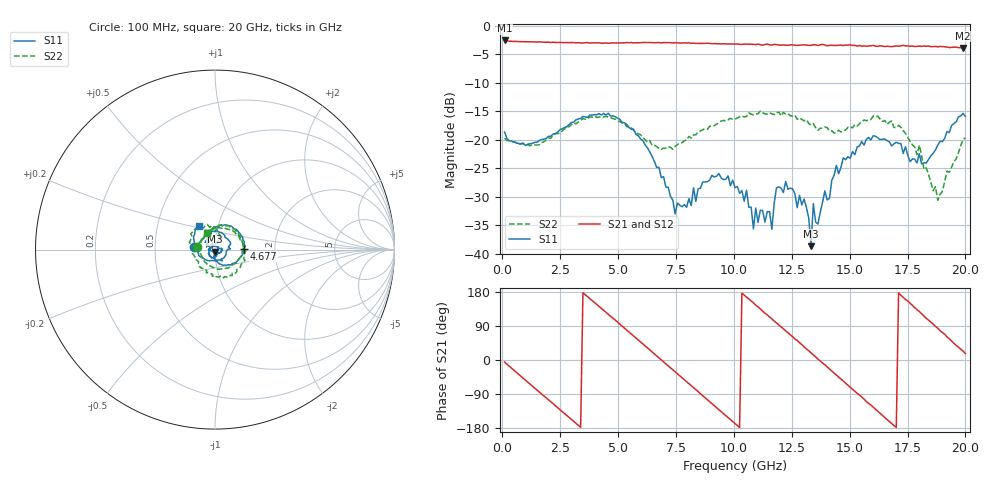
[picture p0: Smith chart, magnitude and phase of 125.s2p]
!Agilent Technologies,N5230C,MY49001569,A.09.33.09
!Agilent N5230C: A.09.33.09
!Date: Tuesday, July 28, 2015 18:46:54
!Correction: S11(Full 2 Port(1,2))
!S21(Full 2 Port(1,2))
!S12(Full 2 Port(1,2))
!S22(Full 2 Port(1,2))
!S2P File: Measurements: S11, S21, S12, S22:
# Hz S  dB  R 50
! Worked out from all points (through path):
!   201 points, 100 MHz to 20 GHz, reference 50 ohm
!   highest |S21| = -2.59 dB at 100 MHz (marker M1); lowest = -3.9 dB at 19.9 GHz (marker M2)
!   group delay of S21, straight-line fit = 147 ps
!   lowest |S11| = -38.7 dB at 13.33 GHz (marker M3), VSWR 1.02, Z = 49.9 - j1.15 ohm
!   |S11| at or under -10 dB: start of sweep to end of sweep
!   |S22| runs from -30.6 to -15.0 dB; largest |S21 - S12| = 0.018
!   S11 on the Smith chart (normalised r, x): 100 MHz: 0.79, +0.03; 4.677 GHz: 1.38, +0.01; 20 GHz: 0.81, +0.22
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1e8  -18.66 172.0  -2.59 -5.4  -2.63 -6.0  -19.74 172.7
1.692e9  -19.97 119.7  -2.88 -89.5  -2.88 -89.4  -20.51 123.6
3.483e9  -15.94 54.6  -3.03 177.5  -3.02 177.6  -16.30 60.3
4.677e9  -15.86 1.8  -3.06 115.4  -3.01 115.7  -16.12 -0.1
5.5725e9  -18.20 -39.7  -2.96 68.9  -2.99 68.9  -17.95 -53.9
6.7665e9  -24.86 -85.3  -2.97 5.8  -2.98 5.8  -21.55 -147.8
7.463e9  -33.02 -89.2  -3.01 -31.1  -3.03 -31.0  -21.17 156.1
8.458e9  -28.61 -86.2  -3.12 -83.4  -3.05 -83.7  -18.65 92.5
1.005e10  -28.44 -151.6  -3.23 -167.8  -3.23 -167.4  -16.40 20.1
1.0846e10  -35.65 149.9  -3.28 150.9  -3.26 150.7  -15.66 -9.4
1.17415e10  -31.18 11.7  -3.27 102.7  -3.29 102.8  -15.63 -42.8
1.3035e10  -30.42 -67.6  -3.36 34.5  -3.35 34.7  -16.69 -88.7
1.33335e10  -38.70 -95.9  -3.45 18.6  -3.36 18.6  -17.45 -107.5
1.3433e10  -31.22 -91.1  -3.34 13.3  -3.52 13.0  -17.21 -110.4
1.3632e10  -34.81 -155.1  -3.49 2.4  -3.44 3.2  -18.35 -116.8
1.5025e10  -23.28 124.6  -3.37 -72.0  -3.45 -70.6  -17.71 -171.3
1.67165e10  -20.38 54.9  -3.65 -162.2  -3.58 -161.9  -16.95 112.1
1.75125e10  -22.75 1.8  -3.54 155.6  -3.57 154.5  -19.63 81.6
1.85075e10  -22.85 -121.2  -3.68 100.3  -3.63 100.3  -27.47 71.8
1.8806e10  -20.97 -152.6  -3.72 83.9  -3.64 84.0  -30.64 91.7
1.99005e10  -15.40 126.6  -3.93 23.5  -3.85 22.1  -19.99 122.0
2e10  -15.94 122.8  -3.92 17.0  -3.92 16.4  -19.69 113.8
